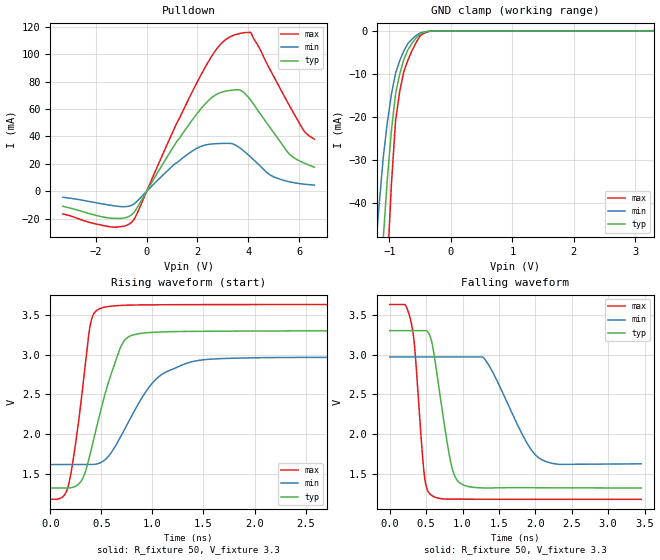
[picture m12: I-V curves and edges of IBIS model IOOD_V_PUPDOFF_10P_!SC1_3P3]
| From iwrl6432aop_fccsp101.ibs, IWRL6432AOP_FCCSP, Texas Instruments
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|   Model Cell IOOD_V_PUPDOFF_10P_!SC1_3P3
|IOOD_V_PUPDOFF_10P_!SC1_3P3
[Model]   IOOD_V_PUPDOFF_10P_!SC1_3P3
Model_type   I/O_open_drain
Polarity   Non-Inverting
Enable   Active-Low
Vinl =  0.8V
Vinh =  2V
Cref =  15pF
Rref =  100.0000M
Vref =  0V
Vmeas =  1.65
|   typ   min   max
C_comp   2.059994p   1.912853p   2.135747p
[Model Spec]
Vinl   0.8V   0.8V   0.8V
Vinh   2V   2V   2V
[Temperature Range]   25   125   -40
[Voltage Range]   3.3   2.97   3.63
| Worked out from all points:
|   slope of the pulldown table from 0 to 0.495 V, typ, clamps not added: 31.8 ohm
|   GND clamp passes 1 mA (typ) near -0.53 V on its own axis
|   rising waveform, R_fixture 50, V_fixture 3.3: 20-80 % time 251ps typ, 385ps min, 143ps max; typ from 1.32 V to 3.3 V
|   falling waveform, R_fixture 50, V_fixture 3.3: 20-80 % time 196ps typ, 423ps min, 118ps max; typ from 3.3 V to 1.32 V
| Where Nom  PVT is Nominal Process, 3.3V, 25C
|   Fast PVT is Strong Process,  3.63V, -40C
|   Slow PVT is Weak Process,   2.97V, 125C
[Pulldown]
|   voltage   I(typ)   I(min)   I(max)
-3.3V     -10.92mA   -4.307mA   -16.45mA
-1.4V     -19.52mA   -10.22mA   -25.94mA
-600mV    -17.22mA   -10.25mA   -22.66mA
1.1V      33.8mA     19.88mA    46.22mA
2.1V      59.3mA     32.44mA    83.48mA
2.9V      71.86mA    34.84mA    107mA
3.5V      73.95mA    33.66mA    114.2mA
4.1V      66.34mA    24.89mA    115.8mA
4.9V      45.33mA    11.53mA    87.2mA
5.6V      27.47mA    7.046mA    63.1mA
6.2V      20.56mA    5.221mA    43.87mA
6.6V      17.6mA     4.555mA    38.05mA
[GND_clamp]
|   voltage   I(typ)   I(min)   I(max)
-3.3V     -787.2mA   -607.8mA   -1.235A
-1.233V   -85.66mA   -52.14mA   -138.8mA
-1.167V   -66.47mA   -40.37mA   -107.7mA
-1.1V     -48.25mA   -29.37mA   -77.98mA
-1.033V   -34.27mA   -21.19mA   -54.56mA
-966.7mV  -23.06mA   -14.66mA   -35.51mA
-900mV    -14.61mA   -9.789mA   -20.83mA
-833.3mV  -10.05mA   -6.934mA   -14.15mA
-700mV    -4.416mA   -2.931mA   -6.81mA
-500mV    -621.6uA   -443.4uA   -1.094mA
-300mV    -17.13uA   -24.29uA   -23.57uA
3.3V      4.589uA    110.6uA    5.608uA
[Ramp]
| variable   typ   min   max
dV/dt_f  1.1959433/0.19777536n 0.83580782/0.43959778n  1.4762235/0.11853739n
dV/dt_r  1.1917531/0.2345539n 0.82901977/0.48916151n  1.4908433/0.13717949n
R_load = 50
[Rising Waveform]
R_fixture = 50
V_fixture = 3.3
V_fixture_min = 2.97
V_fixture_max = 3.63
|   time   V(typ)   V(min)   V(max)
0s        1.322V     1.617V     1.18V
178.4ps   1.322V     1.617V     1.36V
305.5ps   1.415V     1.617V     2.455V
387.2ps   1.732V     1.617V     3.341V
470.7ps   2.178V     1.631V     3.569V
684.6ps   3.081V     1.957V     3.618V
811.7ps   3.248V     2.264V     3.623V
1.057ns   3.283V     2.716V     3.626V
1.417ns   3.292V     2.919V     3.628V
3.453ns   3.299V     2.966V     3.63V
[Falling Waveform]
R_fixture = 50
V_fixture = 3.3
V_fixture_min = 2.97
V_fixture_max = 3.63
|   time   V(typ)   V(min)   V(max)
0s        3.301V     2.97V      3.629V
295.6ps   3.301V     2.97V      3.399V
346.7ps   3.301V     2.97V      3.046V
475.6ps   3.301V     2.97V      1.483V
569.4ps   3.187V     2.97V      1.232V
833.3ps   1.664V     2.97V      1.181V
967.5ps   1.383V     2.97V      1.181V
1.307ns   1.322V     2.939V     1.181V
2.078ns   1.325V     1.683V     1.179V
3.453ns   1.322V     1.626V     1.179V
